(* Logix 5000 Rung export; software revision 16.03 *)

TYPE MNETRETHERNETTYPE :   // Allows read/write Ethernet settings between the module and processor
STRUCT
   Read : BOOL;   // Enable Ethernet configuration transfer from module to processor
   Write : BOOL;   // Enable Ethernet configuration transfer from processor to module
   Config : MNETRETHERNET;
END_STRUCT
END_TYPE

TYPE MNETRETHERNET :   // Stores the MVI56E-MNETR IP settings
STRUCT
   IP : INT[4];
   Netmask : INT[4];
   Gateway : INT[4];
END_STRUCT
END_TYPE

TYPE MNETRCLOCKTYPE :   // Allows read/write of clock value between the module and processor
STRUCT
   Read : BOOL;   // Reads current time from the module
   Write : BOOL;   // Writes current time from the module
   Config : MNETRDATETIME;   // Date and time configuration read or written between the module and processor
END_STRUCT
END_TYPE

TYPE MNETRDATETIME :   // Stores the date and time value
STRUCT
   Year : DINT;
   Month : DINT;
   Day : DINT;
   Hour : DINT;
   Minute : DINT;
   Seconds : DINT;
END_STRUCT
END_TYPE

ADD_ON_INSTRUCTION AOI56EMNETR_OPTIONAL   (* revision 1.0 *)
// MVI56E-MNETR Optional Add-On Ethernet/Clock
// Revision note:
// Release
VAR_IN_OUT
   MVI56EMNETREthernet : MNETRETHERNETTYPE; {required}   // MVI56E-MCM Rev2 Ethernet Settings
   MVI56EMNETRClock : MNETRCLOCKTYPE; {required}   // MVI56E-MCM Rev2 Clock Settings
   ReadEthernetMSG : MESSAGE; {required}   // Read Ethernet Settings Message
   WriteEthernetMSG : MESSAGE; {required}   // Write Ethernet Settings Message
   ReadClockMSG : MESSAGE; {required}   // Read Clock Settings Message
   WriteClockMSG : MESSAGE; {required}   // Write Clock Settings Message
END_VAR

ROUTINE Logic   (* ladder *)
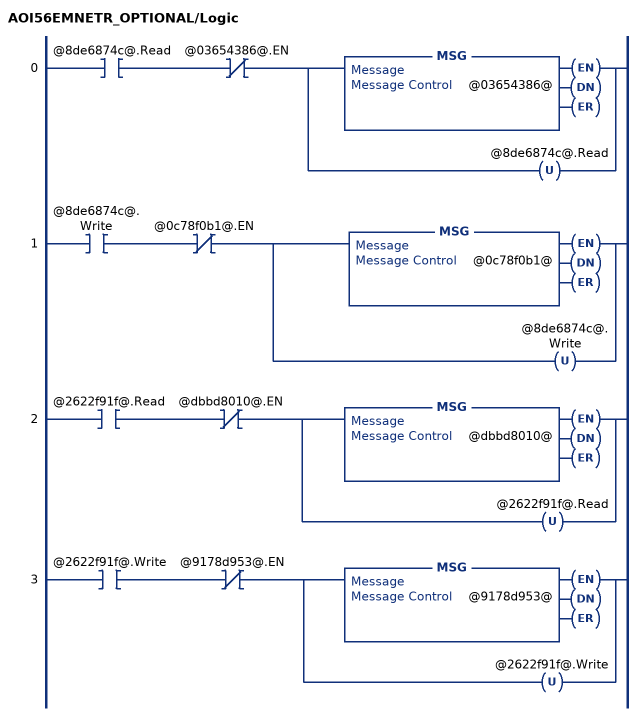
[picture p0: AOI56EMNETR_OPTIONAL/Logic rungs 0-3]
   0: XIC(@8de6874c@.Read)XIO(@03654386@.EN)[MSG(@03654386@) ,OTU(@8de6874c@.Read) ];
   1: XIC(@8de6874c@.Write)XIO(@0c78f0b1@.EN)[MSG(@0c78f0b1@) ,OTU(@8de6874c@.Write) ];
   2: XIC(@2622f91f@.Read)XIO(@dbbd8010@.EN)[MSG(@dbbd8010@) ,OTU(@2622f91f@.Read) ];
   3: XIC(@2622f91f@.Write)XIO(@9178d953@.EN)[MSG(@9178d953@) ,OTU(@2622f91f@.Write) ];
END_ROUTINE
END_ADD_ON_INSTRUCTION

VAR_GLOBAL   (* controller tags *)
   MVI56EMNETRClock : MNETRCLOCKTYPE;
   ReadClockMSG : MESSAGE;
        MessageParameters(MessageType := CIP Generic, ConnectedFlag := 2, ConnectionPath := MNETR, ServiceCode := 16#000e, ObjectType := 16#0004, TargetObject := 8, AttributeNumber := 16#0020, DestinationTag := MVI56EMNETRClock.Config)
   WriteEthernetMSG : MESSAGE;
        MessageParameters(MessageType := CIP Generic, RequestedLength := 24, ConnectedFlag := 2, ConnectionPath := MNETR, ServiceCode := 16#0010, ObjectType := 16#0004, TargetObject := 8, LocalElement := MVI56EMNETREthernet.Config)
   ReadEthernetMSG : MESSAGE;
        MessageParameters(MessageType := CIP Generic, ConnectedFlag := 2, ConnectionPath := MNETR, ServiceCode := 16#000e, ObjectType := 16#0004, TargetObject := 8, DestinationTag := MVI56EMNETREthernet.Config)
   MVI56EMNETREthernet : MNETRETHERNETTYPE;
   WriteClockMSG : MESSAGE;
        MessageParameters(MessageType := CIP Generic, RequestedLength := 24, ConnectedFlag := 2, ConnectionPath := MNETR, ServiceCode := 16#0010, ObjectType := 16#0004, TargetObject := 8, AttributeNumber := 16#0020, LocalElement := MVI56EMNETRClock.Config)
   AOI56EMNETR_Optional : AOI56EMNETR_OPTIONAL;
END_VAR

PROGRAM MainProgram

ROUTINE MainRoutine   (* ladder *)
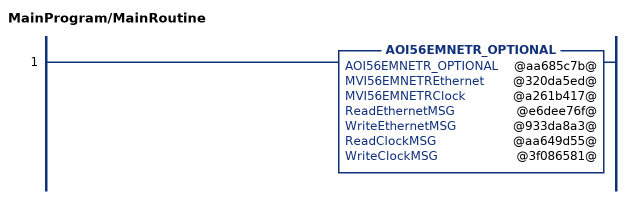
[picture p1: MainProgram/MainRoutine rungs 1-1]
   1: AOI56EMNETR_OPTIONAL(@aa685c7b@,@320da5ed@,@a261b417@,@e6dee76f@,@933da8a3@,@aa649d55@,@3f086581@);
END_ROUTINE
END_PROGRAM
